PROGRAM MAIN
VAR
    Target_x,Target_y: 	LREAL;	// 目标点坐标     
	Distance:			ARRAY[1..3] OF LREAL;	//距离值
END_VAR


	(**********************调用方法********************* *)
	
	// 两点式方法，输入直线上面任意2个点多坐标，以及直线外的P0坐标
	Distance[1] := F_TwoPoints(10, 10, 20, 20, Target_x, Target_y);

	// 一般式方法，根据直线方程系数 Ax + By + C = 0，输入A、B、C的值，以及直线外的P0坐标
	Distance[2] := F_General(0.5, 10, 30, Target_x, Target_y);
	
	// 斜截式方法，根据直线方程 y = kx + b，输入k、b的值，以及直线外的P0坐标
    Distance[3] := F_SlopeIntercept(0.5, 20, Target_x, Target_y);

END_PROGRAM
